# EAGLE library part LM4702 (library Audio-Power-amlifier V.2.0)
The LM4702 is a high fidelity audio power amplifier driver designed for demanding consumer and pro-audio applications. Amplifier output power may be scaled by changing the supply voltage and number of output devices. The LM4702 is capable of delivering in excess of 300 watts per channel single ended into an 8 ohm load in the presence of 10% high line headroom and 20% supply regulation. The LM4702 includes thermal shut down circuitry that activates when the die temperature exceeds 150°C. The LM4702's mute function, when activated, mutes the input drive signal and forces the amplifier output to a quiescent state.
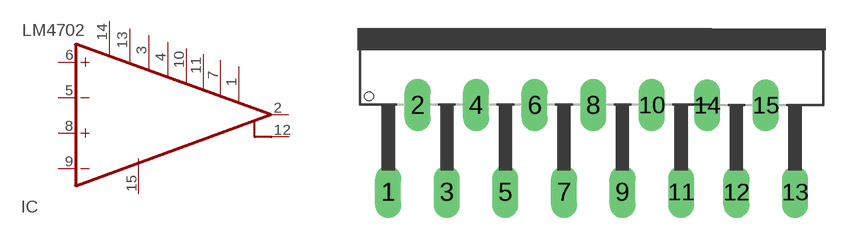
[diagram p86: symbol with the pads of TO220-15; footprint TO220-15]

Designator prefix IC

## LM4702  [TO220-15]
1  V+7  pwr
2  OUT  out
3  V+2  pwr
4  V+3  pwr
5  -INA  in
6  +INA  in
7  V+6  pwr
8  +INB  in
9  -INB  in
10  V+4  pwr
11  V+5  pwr
12  OUT1  out
13  V+  pwr
14  V+1  pwr
15  V-  pwr

## Footprint TO220-15 (pad centres in mm)
drill 1.016 long: 1 0.381,1.905; 2 2.083,6.96; 3 3.785,1.905; 4 5.486,6.96; 5 7.188,1.905; 6 8.89,6.96; 7 10.592,1.905; 8 12.294,6.96; 9 13.995,1.905; 10 15.697,6.96; 11 17.399,1.905; 12 20.615,1.895; 13 24.019,1.895; 14 18.914,6.95; 15 22.317,6.95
